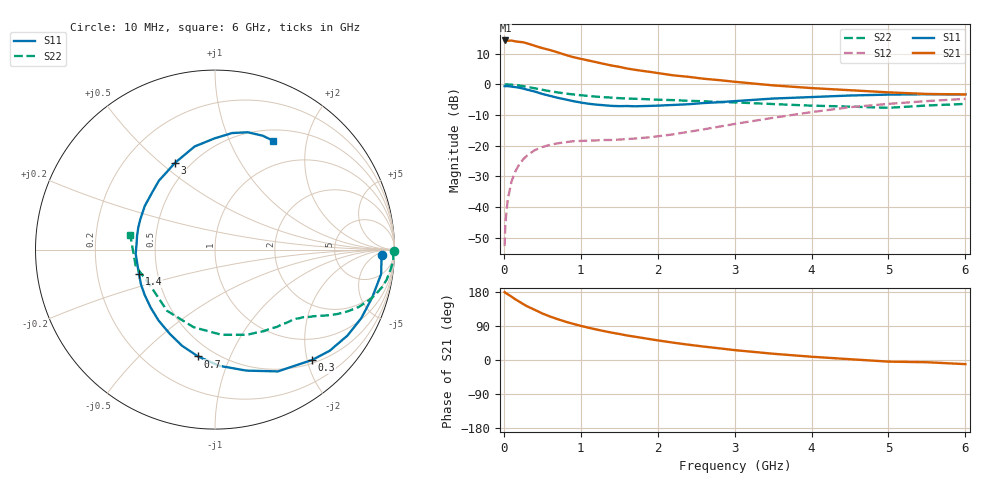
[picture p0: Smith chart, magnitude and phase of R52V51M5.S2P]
! SIEMENS Small Signal Semiconductors
! BFR183
! Si NPN RF Bipolar Junction Transistor in SOT23
! VCE = 2.5 V  IC = 1.5 mA
! Common Emitter S-Parameters:  May  1996
# GHz  S  MA  R  50
!  f  S11  S21  S12  S22
! GHz  MAG  ANG  MAG  ANG  MAG  ANG  MAG  ANG
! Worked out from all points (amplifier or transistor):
!   36 points, 10 MHz to 6 GHz, reference 50 ohm
!   highest |S21| = 14.3 dB at 20 MHz (marker M1)
!   |S21| within 3 dB of that: start of sweep to 578.9 MHz
!   unconditionally stable (mu >= 1): 1.49 GHz to 2.899 GHz
!   at 250 MHz: K = 0.19, MSG = 19.1 dB, |S12| = -24.5 dB
!   at 1.4 GHz: K = 0.96, MSG = 12.1 dB, |S12| = -18.2 dB
!   at 6 GHz: K = 0.93, MSG = 0.7 dB, |S12| = -4.8 dB
!   S11 on the Smith chart (normalised r, x): 10 MHz: 24, -10; 300 MHz: 0.56, -2.09; 700 MHz: 0.41, -0.77; 1.4 GHz: 0.39, -0.13; 3 GHz: 0.41, +0.56; 6 GHz: 0.64, +1.47
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0.01  0.9325 -1.7  5.177 179.1  0.0023 86.3  0.9973 -0.6
0.02  0.929 -3.5  5.182 177.3  0.0053 84.4  0.9923 -1.3
0.05  0.9358 -8.3  5.137 173.6  0.0131 85.7  0.9957 -3.4
0.1  0.9157 -16.9  5.161 167.1  0.0261 80.3  0.9848 -6.4
0.15  0.8999 -25.2  5.007 160.1  0.0382 75.2  0.9716 -9.8
0.25  0.8521 -41.4  4.845 147.8  0.0596 66.4  0.9315 -15.3
0.3  0.8195 -48.6  4.66 142.0  0.0686 62.9  0.9077 -17.8
0.4  0.7636 -62.7  4.249 132.6  0.0841 56.4  0.8618 -21.8
0.5  0.6964 -75.5  3.888 122.8  0.095 50.9  0.815 -25.0
0.6  0.6478 -87.9  3.612 114.8  0.103 46.3  0.7716 -27.7
0.7  0.6028 -99.0  3.316 107.7  0.1091 43.2  0.7374 -29.7
0.8  0.5665 -108.9  3.022 101.2  0.1137 40.6  0.7061 -31.4
0.9  0.5324 -118.3  2.776 95.5  0.118 38.8  0.6846 -32.7
1.1  0.4826 -137.9  2.445 85.2  0.1208 37.3  0.6459 -35.5
1.4  0.4449 -162.2  2.023 72.3  0.1237 38.0  0.6065 -39.1
1.8  0.4412 169.8  1.656 58.3  0.1337 43.3  0.5755 -44.2
2.2  0.4607 148.1  1.4 45.8  0.1527 49.5  0.5524 -51.1
3  0.5317 115.0  1.1 26.1  0.2258 54.5  0.5069 -69.5
3.5  0.5858 101.1  0.96 16.5  0.2844 51.8  0.4763 -85.5
4.5  0.6565 81.6  0.801 2.1  0.4235 39.5  0.433 -128.0
5.5  0.6879 67.3  0.696 -5.9  0.5332 23.9  0.4512 -167.9
6  0.6877 62.0  0.683 -10.9  0.5785 14.4  0.4791 170.2
